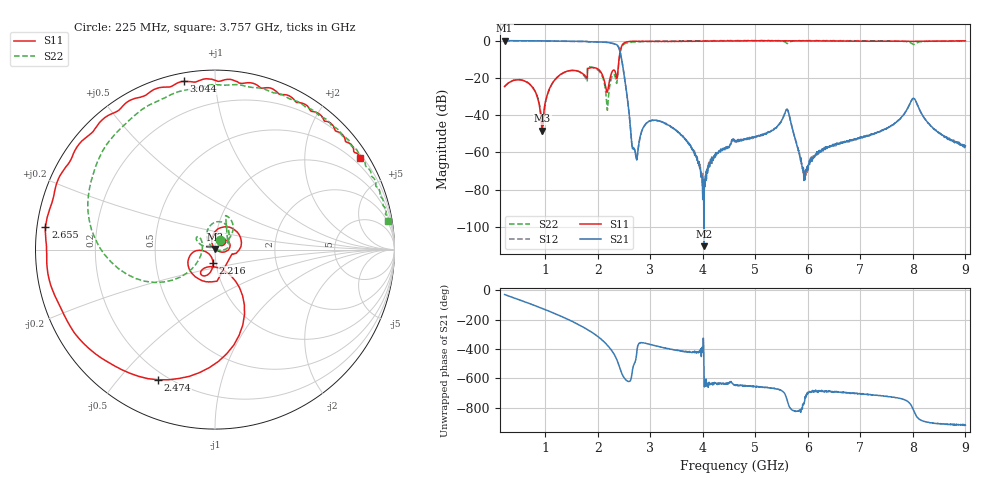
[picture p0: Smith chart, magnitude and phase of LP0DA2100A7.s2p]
!Agilent Technologies,E8358A,US41080443,A.07.50.56
!Agilent E8358A: A.07.50.56
!Date: Tuesday, April 25, 2017 07:57:33
!Correction: S11(Full 2 Port(1,2))
!S21(Full 2 Port(1,2))
!S12(Full 2 Port(1,2))
!S22(Full 2 Port(1,2))
!S2P File: Measurements: S11, S21, S12, S22:
# Hz S  dB  R 50
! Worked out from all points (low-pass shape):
!   1601 points, 225 MHz to 9 GHz, reference 50 ohm
!   highest |S21| = -0.05 dB at 225 MHz (marker M1); lowest = -110.3 dB at 4.02 GHz (marker M2)
!   |S21| within 3 dB of the highest: start of sweep to 2.385 GHz
!   lowest |S11| = -48.4 dB at 943.5 MHz (marker M3), VSWR 1.01, Z = 50.2 + j0.322 ohm
!   |S11| at or under -10 dB: start of sweep to 2.404 GHz
!   |S22| runs from -50.2 to 0.0 dB; largest |S21 - S12| = 0.0093
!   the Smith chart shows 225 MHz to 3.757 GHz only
!   S11 on the Smith chart (normalised r, x): 225 MHz: 1.06, +0.10; 2.216 GHz: 0.97, -0.14; 2.474 GHz: 0.17, -0.64; 2.655 GHz: 0.02, +0.07; 3.044 GHz: 0.04, +0.83; 3.757 GHz: 0.27, +3.43
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2.25e8  -24.70 57.7  -0.05 -29.0  -0.12 -28.8  -24.71 60.8
6.966562e8  -23.30 -5.3  -0.15 -89.8  -0.22 -89.9  -23.19 6.6
9.434531e8  -48.42 57.8  -0.18 -123.7  -0.25 -123.8  -50.21 57.3
1.195734e9  -20.63 93.6  -0.27 -160.6  -0.34 -160.8  -20.75 120.0
1.689328e9  -17.38 0.1  -0.49 116.1  -0.55 115.9  -17.53 55.2
1.963547e9  -14.78 -138.6  -0.72 55.4  -0.78 55.2  -15.07 56.3
2.215828e9  -22.56 -98.9  -1.11 -27.5  -1.19 -27.8  -26.50 162.4
2.336484e9  -17.28 -122.7  -1.95 -92.1  -2.02 -92.3  -20.15 143.3
2.473594e9  -2.03 -113.6  -13.43 141.5  -13.49 141.0  -2.62 163.2
2.654578e9  -0.41 172.3  -57.17 161.6  -57.07 160.4  -0.88 102.6
2.736844e9  -0.43 152.0  -63.57 -80.2  -63.91 -73.6  -0.74 88.2
3.043969e9  -0.41 100.6  -42.83 -12.4  -42.71 -13.5  -0.45 53.7
3.153656e9  -0.50 87.3  -43.08 -22.0  -43.25 -23.3  -0.40 45.3
3.756938e9  -0.36 32.3  -56.12 -60.1  -56.29 -64.6  -0.19 9.5
4.020188e9  -0.30 16.7  -110.34 -138.2  -75.76 43.9  -0.14 -1.3
4.6125e9  -0.21 -7.9  -53.52 76.8  -54.14 74.1  -0.07 -19.9
5.599688e9  -0.20 -33.1  -36.85 -20.2  -36.97 -21.3  -1.54 -44.4
5.917781e9  -0.19 -39.6  -68.63 -58.4  -70.13 -71.7  -0.10 -48.6
6.076828e9  -0.19 -42.6  -64.85 35.5  -63.22 34.9  -0.11 -51.9
7.541156e9  -0.41 -78.9  -46.37 -2.8  -46.47 -5.4  -0.23 -98.2
8.018297e9  -0.48 -90.4  -31.12 -101.0  -31.18 -102.6  -2.15 -110.2
9e9  -0.18 -106.9  -56.51 162.7  -57.01 161.3  -0.43 -132.5
